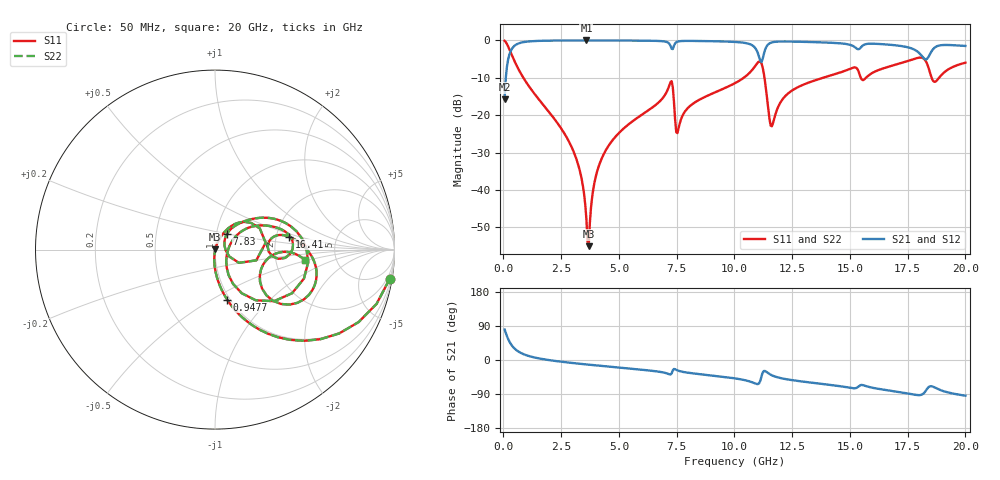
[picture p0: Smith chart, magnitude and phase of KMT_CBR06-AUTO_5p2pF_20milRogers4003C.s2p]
! Data measured by Modelithics Inc. support@modelithics.com 813-866-6335
! KEMET CBR06-AUTO 5.2pF, Pad Width= 0.851mm, Pad Length= 0.64mm, Pad Gap= 0.62mm, 20mil Rogers 4003C substrate Data, January 2022
# hz S ma R 50
! 2 Port Network Data from SP1.SP block
! freq  magS11  angS11  magS21  angS21  magS12  angS12  magS22  angS22
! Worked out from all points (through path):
!   401 points, 50 MHz to 20 GHz, reference 50 ohm
!   highest |S21| = -0.01 dB at 3.591 GHz (marker M1); lowest = -15.8 dB at 50 MHz (marker M2)
!   group delay of S21, straight-line fit = 15.2 ps
!   lowest |S11| = -55.0 dB at 3.691 GHz (marker M3), VSWR 1.00, Z = 50.2 + j0.0627 ohm
!   |S11| at or under -10 dB: 862.3 MHz to 10.4 GHz (9.539 GHz wide, 169 % of centre); 11.3 GHz to 13.84 GHz (2.535 GHz wide, 20.2 % of centre); 18.54 GHz to 18.86 GHz (320.6 MHz wide, 1.71 % of centre)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
!   |S22| runs from -55.0 to -0.1 dB; largest |S21 - S12| = 0
!   S11 on the Smith chart (normalised r, x): 50 MHz: 1, -12; 947.8 MHz: 0.97, -0.59; 7.83 GHz: 1.12, +0.20; 16.41 GHz: 2.36, +0.41; 20 GHz: 2.95, -0.46
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5e7  0.9867 -9.5  0.1625 80.5  0.1625 80.5  0.9867 -9.5
3.4925e8  0.6525 -50.4  0.7571 39.6  0.7571 39.6  0.6525 -50.4
9.4775e8  0.2871 -76.3  0.957 13.5  0.957 13.5  0.2871 -76.3
2.74325e9  0.05017 -94.8  0.9973 -6.3  0.9973 -6.3  0.05017 -94.8
3.391625e9  0.01374 -94.5  0.9984 -10.5  0.9984 -10.5  0.01374 -94.5
3.591125e9  0.004074 -80.6  0.9984 -11.7  0.9984 -11.7  0.004074 -80.6
3.690875e9  0.001775 20.6  0.9984 -12.3  0.9984 -12.3  0.001775 20.6
3.990125e9  0.0148 69.9  0.9982 -14.1  0.9982 -14.1  0.0148 69.9
4.439e9  0.03431 70.5  0.9976 -16.7  0.9976 -16.7  0.03431 70.5
6.73325e9  0.1496 56.7  0.9823 -30.9  0.9823 -30.9  0.1496 56.7
7.232e9  0.276 25.5  0.8463 -38.2  0.8463 -38.2  0.276 25.5
7.53125e9  0.05763 22.8  0.9619 -27.4  0.9619 -27.4  0.05763 22.8
7.8305e9  0.1088 52.6  0.9838 -32.1  0.9838 -32.1  0.1088 52.6
1.0025e10  0.2682 39.5  0.9536 -48.5  0.9536 -48.5  0.2682 39.5
1.112225e10  0.5213 -18.0  0.5311 -54.5  0.5311 -54.5  0.5213 -18.0
1.1621e10  0.07121 -5.7  0.9402 -40.3  0.9402 -40.3  0.07121 -5.7
1.336662e10  0.2839 28.3  0.9501 -60.0  0.9501 -60.0  0.2839 28.3
1.6409e10  0.4192 9.9  0.8904 -77.8  0.8904 -77.8  0.4192 9.9
1.670825e10  0.448 7.3  0.8763 -80.5  0.8763 -80.5  0.448 7.3
1.830425e10  0.516 -36.4  0.5579 -79.4  0.5579 -79.4  0.516 -36.4
1.870325e10  0.2808 -17.4  0.8151 -73.5  0.8151 -73.5  0.2808 -17.4
2e10  0.5036 -6.6  0.8425 -94.2  0.8425 -94.2  0.5036 -6.6
